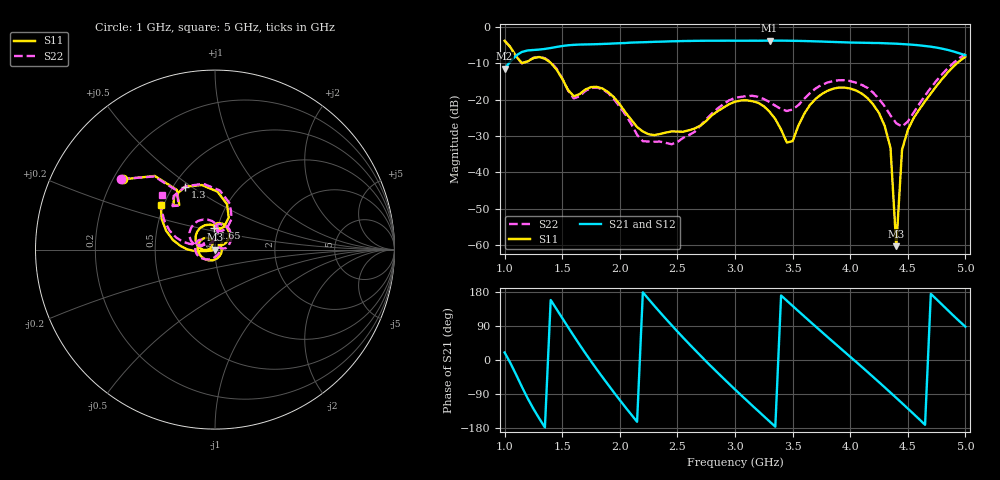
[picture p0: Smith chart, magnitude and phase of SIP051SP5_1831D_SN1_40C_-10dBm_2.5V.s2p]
# GHz  S  dB  R  50
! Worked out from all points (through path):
!   81 points, 1 GHz to 5 GHz, reference 50 ohm
!   highest |S21| = -3.73 dB at 3.3 GHz (marker M1); lowest = -11.4 dB at 1 GHz (marker M2)
!   lowest |S11| = -60.3 dB at 4.4 GHz (marker M3), VSWR 1.00, Z = 49.9 + j0.0191 ohm
!   |S11| at or under -10 dB: 1.405 GHz to 4.926 GHz (3.521 GHz wide, 111 % of centre)
!   |S22| runs from -32.3 to -3.7 dB; largest |S21 - S12| = 0.0022
!   S11 on the Smith chart (normalised r, x): 1 GHz: 0.24, +0.32; 1.3 GHz: 0.57, +0.47; 1.65 GHz: 0.96, +0.23; 5 GHz: 0.48, +0.28
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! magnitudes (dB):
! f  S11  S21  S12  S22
! 1 GHz  -3.8  -11.4  -11.4  -3.7
! 1.15 GHz  -9.9  -6.8  -6.8  -10.0
! 1.3 GHz  -8.2  -6.2  -6.2  -8.2
! 1.65 GHz  -18.5  -4.8  -4.8  -19.1
! 1.7 GHz  -17.2  -4.8  -4.8  -17.6
! 1.85 GHz  -16.9  -4.6  -4.6  -17.1
! 2.2 GHz  -28.8  -4.2  -4.2  -31.4
! 2.35 GHz  -29.4  -4.0  -4.0  -31.5
! 2.5 GHz  -28.8  -3.9  -3.9  -31.7
! 3 GHz  -20.6  -3.8  -3.7  -19.5
! 3.3 GHz  -23.3  -3.7  -3.7  -20.6
! 3.45 GHz  -31.8  -3.7  -3.8  -23.1
! 3.5 GHz  -31.4  -3.8  -3.8  -22.7
! 3.7 GHz  -19.8  -3.9  -3.9  -16.9
! 3.9 GHz  -16.7  -4.1  -4.2  -14.6
! 4.1 GHz  -18.3  -4.3  -4.3  -15.9
! 4.25 GHz  -23.7  -4.4  -4.4  -19.8
! 4.35 GHz  -33.3  -4.5  -4.5  -24.3
! 4.4 GHz  -60.3  -4.6  -4.6  -26.5
! 4.45 GHz  -33.8  -4.7  -4.7  -27.4
! 4.5 GHz  -28.3  -4.8  -4.8  -26.0
! 5 GHz  -8.2  -7.8  -7.8  -7.4
